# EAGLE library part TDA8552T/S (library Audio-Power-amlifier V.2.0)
2 ´ 1.4 W BTL audio amplifiers with digital volume control and headphone sensing
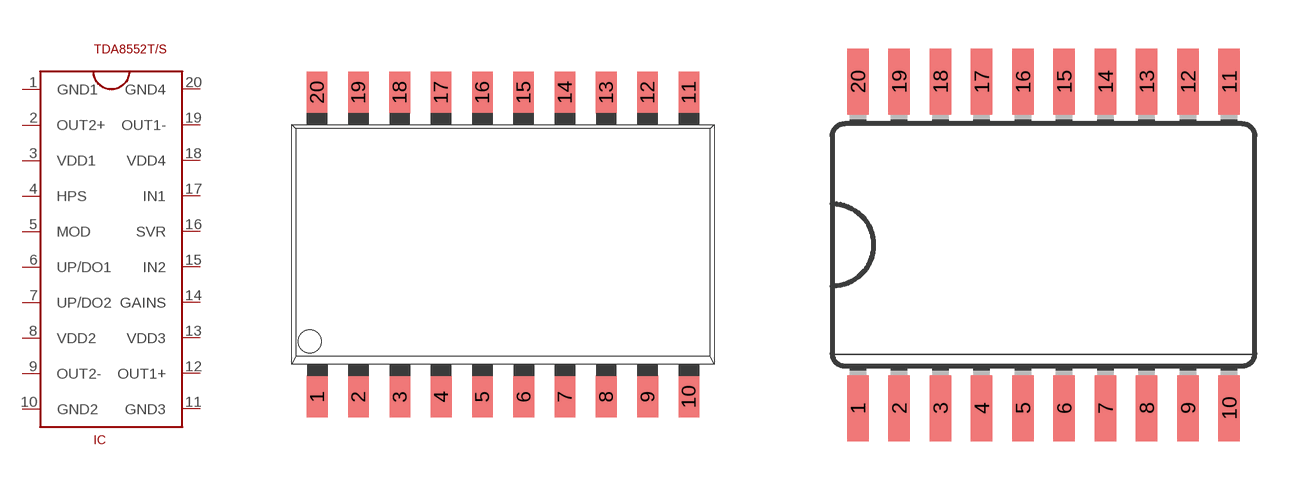
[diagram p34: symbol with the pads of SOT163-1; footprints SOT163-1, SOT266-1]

Designator prefix IC

## TDA8552T/S  [SOT163-1]
1  GND1  pwr
2  OUT2+  out
3  VDD1  pwr
4  HPS
5  MOD
6  UP/DO1
7  UP/DO2
8  VDD2  pwr
9  OUT2-  out
10  GND2  pwr
11  GND3  pwr
12  OUT1+  out
13  VDD3  pwr
14  GAINS
15  IN2  in
16  SVR
17  IN1  in
18  VDD4  pwr
19  OUT1-  out
20  GND4  pwr

## TDA8552T/SSOT266-1  [SOT266-1]
Pads as for SOT163-1

## Footprint SOT163-1 (pad centres in mm)
smd 0.635 x 1.27: 1 -5.71,-4.685; 2 -4.445,-4.685; 3 -3.17,-4.685; 4 -1.9,-4.685; 5 -0.635,-4.685; 6 0.64,-4.685; 7 1.905,-4.685; 8 3.175,-4.685; 9 4.45,-4.685; 10 5.715,-4.685; 11 5.715,4.685; 12 4.445,4.685; 13 3.175,4.685; 14 1.905,4.685; 15 0.635,4.685; 16 -0.635,4.685; 17 -1.905,4.685; 18 -3.175,4.685; 19 -4.445,4.685; 20 -5.715,4.685

## Footprint SOT266-1 (pad centres in mm)
Small Outline Package
smd 0.66 x 2.032: 1 -5.715,-5.029; 2 -4.445,-5.029; 3 -3.175,-5.029; 4 -1.905,-5.029; 5 -0.635,-5.029; 6 0.635,-5.029; 7 1.905,-5.029; 8 3.175,-5.029; 9 4.445,-5.029; 10 5.715,-5.029; 11 5.715,5.029; 12 4.445,5.029; 13 3.175,5.029; 14 1.905,5.029; 15 0.635,5.029; 16 -0.635,5.029; 17 -1.905,5.029; 18 -3.175,5.029; 19 -4.445,5.029; 20 -5.715,5.029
